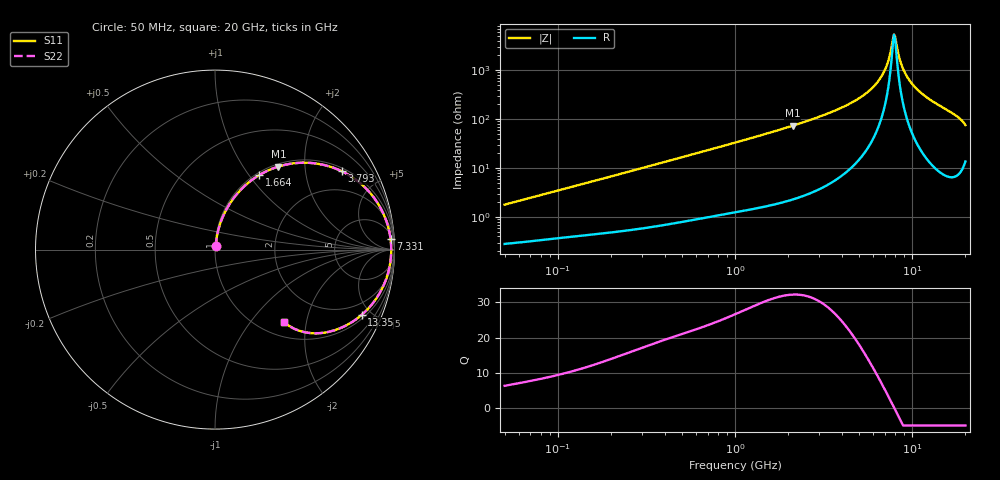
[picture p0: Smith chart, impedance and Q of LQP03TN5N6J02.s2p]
!Murata Part Number: LQP03TN5N6J02
!These Parameters are Measured in Series Mode Connection
!  o--[Z]--o
!Port1  Port2
!  o-------o
!Freq. Start=50[MHz] Stop=20[GHz], 401[Steps]
# Hz S RI R 50
!Freq.(Hz) S11(Real) S11(Imag) S21(Real) S21(Imag) S12(Real) S12(Imag) S22(Real) S22(Imag)
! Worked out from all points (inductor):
!   401 points, 50 MHz to 20 GHz, reference 50 ohm
!   read as one part in series: L = 5.57 nH near 51.52 MHz
!   highest Q = 32.2 at 2.115 GHz (marker M1), where L = 5.51 nH
!   self-resonance near 7.902 GHz
!   S11 on the Smith chart (normalised r, x): 50 MHz: 1.01, +0.04; 1.664 GHz: 1.04, +1.12; 3.793 GHz: 1.12, +3.15; 7.331 GHz: 10, +29; 13.35 GHz: 1.21, -4.39; 20 GHz: 1.27, -1.48
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5e7  0.00311 0.0175  0.9969 -0.0175  0.9969 -0.0175  0.00311 0.0175
1.364002e8  0.00626 0.046  0.9937 -0.046  0.9937 -0.046  0.00626 0.046
3.721004e8  0.0213 0.1204  0.9787 -0.1204  0.9787 -0.1204  0.0213 0.1204
1e9  0.1073 0.2913  0.8927 -0.2913  0.8927 -0.2913  0.1073 0.2913
1.664083e9  0.2468 0.4154  0.7532 -0.4154  0.7532 -0.4154  0.2468 0.4154
2.114743e9  0.3537 0.4629  0.6463 -0.4629  0.6463 -0.4629  0.3537 0.4629
2.728004e9  0.4969 0.4843  0.5031 -0.4843  0.5031 -0.4843  0.4969 0.4843
3.792786e9  0.7054 0.4371  0.2946 -0.4371  0.2946 -0.4371  0.7054 0.4371
4.81993e9  0.8437 0.3382  0.1563 -0.3382  0.1563 -0.3382  0.8437 0.3382
5.856089e9  0.9278 0.2217  0.0722 -0.2217  0.0722 -0.2217  0.9278 0.2217
6.701223e9  0.9647 0.1271  0.0353 -0.1271  0.0353 -0.1271  0.9647 0.1271
7.009217e9  0.9726 0.0939  0.0274 -0.0939  0.0274 -0.0939  0.9726 0.0939
7.331367e9  0.9781 0.06  0.0219 -0.06  0.0219 -0.06  0.9781 0.06
7.442007e9  0.9794 0.0486  0.0206 -0.0486  0.0206 -0.0486  0.9794 0.0486
7.784049e9  0.9817 0.0142  0.0183 -0.0142  0.0183 -0.0142  0.9817 0.0142
8.020766e9  0.9819 -0.00882  0.0181 0.00882  0.0181 0.00882  0.9819 -0.00882
8.644534e9  0.9775 -0.0665  0.0225 0.0665  0.0225 0.0665  0.9775 -0.0665
9.457416e9  0.9631 -0.1348  0.0369 0.1348  0.0369 0.1348  0.9631 -0.1348
1.082228e10  0.9229 -0.2326  0.0771 0.2326  0.0771 0.2326  0.9229 -0.2326
1.334722e10  0.8172 -0.3638  0.1828 0.3638  0.1828 0.3638  0.8172 -0.3638
1.747767e10  0.5923 -0.4647  0.4077 0.4647  0.4077 0.4647  0.5923 -0.4647
2e10  0.3828 -0.4029  0.6172 0.4029  0.6172 0.4029  0.3828 -0.4029
